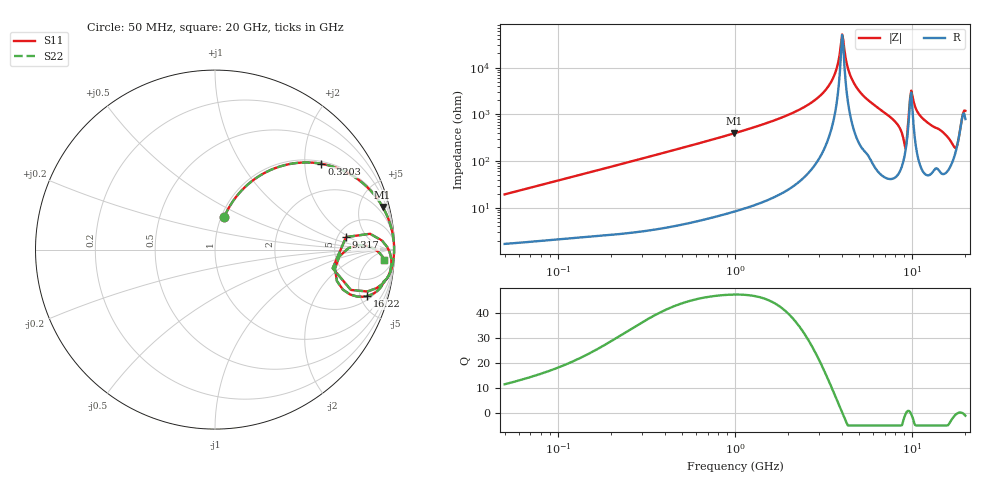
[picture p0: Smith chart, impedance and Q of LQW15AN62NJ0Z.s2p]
!Murata Part Number: LQW15AN62NJ0Z
!These Parameters are Measured in Series Mode Connection
!  o--[Z]--o
!Port1  Port2
!  o-------o
!Freq. Start=50[MHz] Stop=20[GHz], 401[Steps]
# Hz S RI R 50
!Freq.(Hz) S11(Real) S11(Imag) S21(Real) S21(Imag) S12(Real) S12(Imag) S22(Real) S22(Imag)
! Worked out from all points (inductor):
!   401 points, 50 MHz to 20 GHz, reference 50 ohm
!   read as one part in series: L = 61.2 nH near 51.52 MHz
!   highest Q = 47.3 at 985.1 MHz (marker M1), where L = 63 nH
!   self-resonance near 4.027 GHz
!   S11 on the Smith chart (normalised r, x): 50 MHz: 1.03, +0.39; 320.3 MHz: 1.06, +2.43; 9.317 GHz: 5.95, +1.80; 16.22 GHz: 2.38, -5.74; 20 GHz: 17, -18
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5e7  0.0509 0.1803  0.9491 -0.1803  0.9491 -0.1803  0.0509 0.1803
1.364002e8  0.2222 0.3939  0.7778 -0.3939  0.7778 -0.3939  0.2222 0.3939
3.203381e8  0.593 0.4781  0.407 -0.4781  0.407 -0.4781  0.593 0.4781
3.721004e8  0.6617 0.4608  0.3383 -0.4608  0.3383 -0.4608  0.6617 0.4608
9.85133e8  0.9338 0.2383  0.0662 -0.2383  0.0662 -0.2383  0.9338 0.2383
1e9  0.9358 0.2348  0.0642 -0.2348  0.0642 -0.2348  0.9358 0.2348
2.728004e9  0.995 0.0544  0.00504 -0.0544  0.00504 -0.0544  0.995 0.0544
3.519108e9  0.9977 0.019  0.00226 -0.019  0.00226 -0.019  0.9977 0.019
3.736399e9  0.998 0.0108  0.00201 -0.0108  0.00201 -0.0108  0.998 0.0108
4.026975e9  0.9981 0.000415  0.00192 -0.000415  0.00192 -0.000415  0.9981 0.000415
4.405649e9  0.9979 -0.0122  0.00215 0.0122  0.00215 0.0122  0.9979 -0.0122
4.81993e9  0.9972 -0.0253  0.00284 0.0253  0.00284 0.0253  0.9972 -0.0253
7.442007e9  0.983 -0.1082  0.017 0.1082  0.017 0.1082  0.983 -0.1082
8.516016e9  0.9435 -0.1797  0.0565 0.1797  0.0565 0.1797  0.9435 -0.1797
9.041845e9  0.7569 -0.2246  0.2431 0.2246  0.2431 0.2246  0.7569 -0.2246
9.316812e9  0.7303 0.0699  0.2697 -0.0699  0.2697 -0.0699  0.7303 0.0699
9.745021e9  0.9591 0.0147  0.0409 -0.0147  0.0409 -0.0147  0.9591 0.0147
1.004137e10  0.9783 -0.0326  0.0217 0.0326  0.0217 0.0326  0.9783 -0.0326
1.131968e10  0.978 -0.1124  0.022 0.1124  0.022 0.1124  0.978 -0.1124
1.621653e10  0.8477 -0.2586  0.1523 0.2586  0.1523 0.2586  0.8477 -0.2586
1.774144e10  0.6683 -0.107  0.3317 0.107  0.3317 0.107  0.6683 -0.107
2e10  0.9434 -0.0562  0.0566 0.0562  0.0566 0.0562  0.9434 -0.0562
